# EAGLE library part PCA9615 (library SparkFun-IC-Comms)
Differential I2C Bus Buffer Datasheet
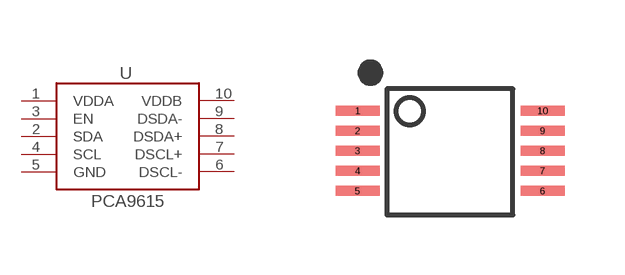
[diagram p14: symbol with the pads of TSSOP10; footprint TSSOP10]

Designator prefix -

## PCA9615 (PROD_ID: IC-13899)  [TSSOP10]
1  VDDA
2  SDA
3  EN
4  SCL
5  GND
6  DSCL-
7  DSCL+
8  DSDA+
9  DSDA-
10  VDDB

## Footprint TSSOP10 (pad centres in mm)
smd 1.1 x 0.25: 1 -2.259,1.018; 2 -2.259,0.517; 3 -2.259,0.018; 4 -2.259,-0.482; 5 -2.259,-0.988; 6 2.366,-0.988; 7 2.366,-0.482; 8 2.366,0.018; 9 2.366,0.517; 10 2.366,1.018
